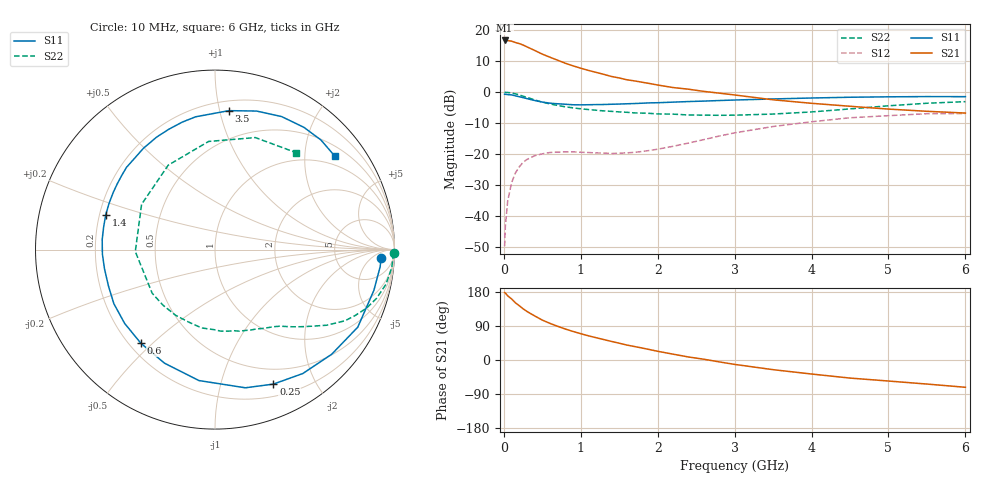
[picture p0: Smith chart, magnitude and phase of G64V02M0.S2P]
! SIEMENS Small Signal Semiconductors
! BFG193
! Si NPN RF Bipolar Junction Transistor in SOT223
! VCE = 4 V  IC = 2 mA
! Common Emitter S-Parameters:  August  1996
# GHz  S  MA  R  50
!  f  S11  S21  S12  S22
! GHz  MAG  ANG  MAG  ANG  MAG  ANG  MAG  ANG
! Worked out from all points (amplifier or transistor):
!   36 points, 10 MHz to 6 GHz, reference 50 ohm
!   highest |S21| = 16.7 dB at 10 MHz (marker M1)
!   |S21| within 3 dB of that: start of sweep to 382.2 MHz
!   unconditionally stable (mu >= 1): 1.364 GHz to 2.571 GHz
!   at 250 MHz: K = 0.18, MSG = 18.9 dB, |S12| = -22.6 dB
!   at 1.4 GHz: K = 1.03, MAG = 11.3 dB, |S12| = -19.8 dB
!   at 6 GHz: K = 0.95, MSG = 0.1 dB, |S12| = -6.9 dB
!   S11 on the Smith chart (normalised r, x): 10 MHz: 19, -12; 250 MHz: 0.33, -1.47; 600 MHz: 0.25, -0.46; 1.4 GHz: 0.23, +0.15; 3.5 GHz: 0.27, +1.07; 6 GHz: 0.74, +2.73
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0.01  0.9258 -2.8  6.818 177.8  0.0033 90.1  0.9967 -1.2
0.02  0.9252 -5.9  6.789 176.8  0.007 88.2  0.9927 -2.4
0.05  0.9139 -14.4  6.781 169.4  0.0176 82.1  0.9899 -5.8
0.1  0.9053 -28.5  6.642 161.3  0.0346 75.2  0.9719 -11.5
0.15  0.8733 -41.9  6.318 151.0  0.0498 66.3  0.9399 -16.8
0.2  0.8461 -54.7  6.075 143.3  0.0625 60.6  0.9054 -21.1
0.25  0.817 -66.5  5.755 135.2  0.0739 53.8  0.8619 -25.3
0.3  0.7883 -77.6  5.378 128.2  0.0823 49.0  0.8257 -28.7
0.4  0.7351 -97.0  4.715 116.4  0.0945 40.3  0.7516 -34.1
0.5  0.6925 -114.0  4.105 105.3  0.1016 33.3  0.6913 -38.1
0.6  0.6653 -128.4  3.658 96.6  0.1067 28.6  0.647 -41.6
0.8  0.6391 -151.9  2.924 81.7  0.1092 21.8  0.5809 -47.5
0.9  0.6272 -161.3  2.657 75.3  0.1092 19.9  0.5587 -49.8
1.1  0.6279 -177.8  2.243 63.8  0.1066 18.5  0.5243 -56.1
1.4  0.639 162.2  1.791 49.0  0.1028 20.1  0.4909 -65.8
1.6  0.6503 150.7  1.584 39.4  0.1053 23.6  0.4743 -73.3
2.2  0.6914 125.1  1.188 15.4  0.1343 33.3  0.4428 -99.7
2.8  0.7336 104.3  0.965 -5.0  0.1964 31.8  0.4241 -133.1
3.5  0.778 84.3  0.754 -25.5  0.2799 17.6  0.4442 -178.6
4.5  0.8289 63.4  0.593 -47.7  0.3871 -6.9  0.5377 119.0
5.5  0.8493 46.0  0.492 -63.5  0.4501 -36.1  0.6634 70.2
6  0.8467 37.9  0.461 -72.0  0.4519 -51.5  0.7038 50.2
